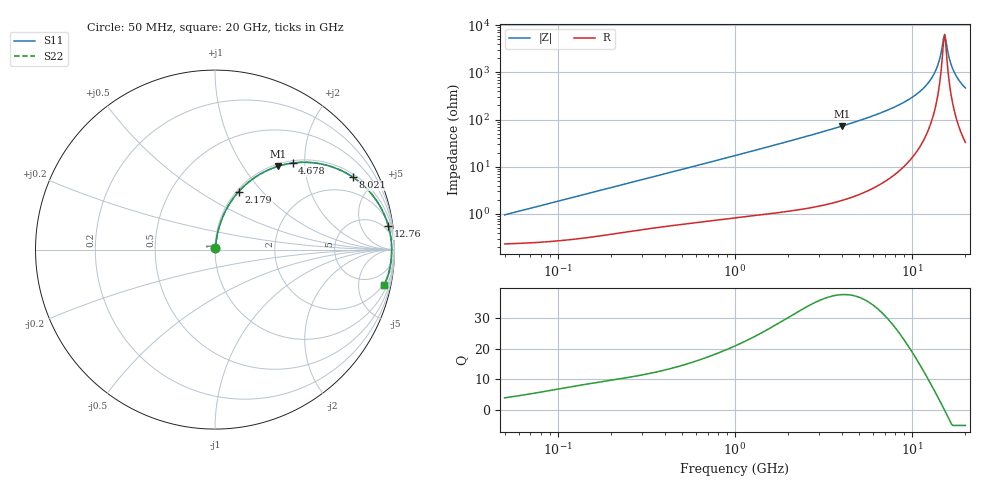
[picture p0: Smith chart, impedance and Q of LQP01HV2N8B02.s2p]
!Murata Part Number: LQP01HV2N8B02
!These Parameters are Measured in Series Mode Connection
!  o--[Z]--o
!Port1  Port2
!  o-------o
!Freq. Start=50[MHz] Stop=20[GHz], 401[Steps]
# Hz S RI R 50
!Freq.(Hz) S11(Real) S11(Imag) S21(Real) S21(Imag) S12(Real) S12(Imag) S22(Real) S22(Imag)
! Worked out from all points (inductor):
!   401 points, 50 MHz to 20 GHz, reference 50 ohm
!   read as one part in series: L = 2.95 nH near 51.52 MHz
!   highest Q = 37.7 at 4.027 GHz (marker M1), where L = 2.88 nH
!   self-resonance near 15.05 GHz
!   S11 on the Smith chart (normalised r, x): 50 MHz: 1.00, +0.02; 2.179 GHz: 1.02, +0.75; 4.678 GHz: 1.05, +1.74; 8.021 GHz: 1.14, +3.72; 12.76 GHz: 3, +14; 20 GHz: 1.66, -9.30
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5e7  0.0024 0.00925  0.9976 -0.00925  0.9976 -0.00925  0.0024 0.00925
1.364002e8  0.00366 0.0248  0.9963 -0.0248  0.9963 -0.0248  0.00366 0.0248
3.721004e8  0.00942 0.0648  0.9906 -0.0648  0.9906 -0.0648  0.00942 0.0648
1e9  0.0362 0.1644  0.9638 -0.1644  0.9638 -0.1644  0.0362 0.1644
2.179053e9  0.1318 0.3228  0.8682 -0.3228  0.8682 -0.3228  0.1318 0.3228
2.728004e9  0.1915 0.3793  0.8085 -0.3793  0.8085 -0.3793  0.1915 0.3793
4.026975e9  0.3509 0.4642  0.6491 -0.4642  0.6491 -0.4642  0.3509 0.4642
4.677679e9  0.4322 0.4822  0.5678 -0.4822  0.5678 -0.4822  0.4322 0.4822
7.442007e9  0.7227 0.4308  0.2773 -0.4308  0.2773 -0.4308  0.7227 0.4308
8.020766e9  0.7682 0.4038  0.2318 -0.4038  0.2318 -0.4038  0.7682 0.4038
1.066139e10  0.9113 0.2554  0.0887 -0.2554  0.0887 -0.2554  0.9113 0.2554
1.276073e10  0.9655 0.1328  0.0345 -0.1328  0.0345 -0.1328  0.9655 0.1328
1.375312e10  0.9779 0.0778  0.0221 -0.0778  0.0221 -0.0778  0.9779 0.0778
1.417136e10  0.9811 0.0554  0.0189 -0.0554  0.0189 -0.0554  0.9811 0.0554
1.482269e10  0.9839 0.0215  0.0161 -0.0215  0.0161 -0.0215  0.9839 0.0215
1.504638e10  0.9843 0.0102  0.0157 -0.0102  0.0157 -0.0102  0.9843 0.0102
1.527346e10  0.9845 -0.00108  0.0155 0.00108  0.0155 0.00108  0.9845 -0.00108
1.550395e10  0.9844 -0.0124  0.0156 0.0124  0.0156 0.0124  0.9844 -0.0124
1.646126e10  0.9813 -0.0576  0.0187 0.0576  0.0187 0.0576  0.9813 -0.0576
1.721783e10  0.9763 -0.0912  0.0237 0.0912  0.0237 0.0912  0.9763 -0.0912
1.855685e10  0.9628 -0.146  0.0372 0.146  0.0372 0.146  0.9628 -0.146
2e10  0.9432 -0.1988  0.0568 0.1988  0.0568 0.1988  0.9432 -0.1988
